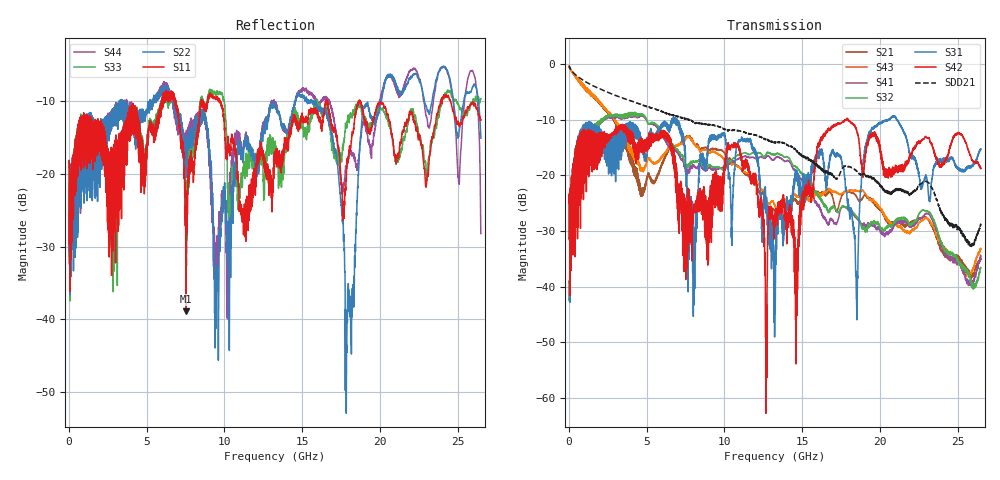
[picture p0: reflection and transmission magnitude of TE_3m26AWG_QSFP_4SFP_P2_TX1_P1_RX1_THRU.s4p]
!Agilent Technologies,N5222A,MY51421691,A.10.00.00
!Agilent N5222A: A.10.00.00
!Date: Friday, January 30, 2015 12:33:28
!Correction: S11(Full 4 Port(1,2,3,4))
!S12(Full 4 Port(1,2,3,4))
!S13(Full 4 Port(1,2,3,4))
!S14(Full 4 Port(1,2,3,4))
!S21(Full 4 Port(1,2,3,4))
!S22(Full 4 Port(1,2,3,4))
!S23(Full 4 Port(1,2,3,4))
!S24(Full 4 Port(1,2,3,4))
!S31(Full 4 Port(1,2,3,4))
!S32(Full 4 Port(1,2,3,4))
!S33(Full 4 Port(1,2,3,4))
!S34(Full 4 Port(1,2,3,4))
!S41(Full 4 Port(1,2,3,4))
!S42(Full 4 Port(1,2,3,4))
!S43(Full 4 Port(1,2,3,4))
!S44(Full 4 Port(1,2,3,4))
!S4P File: Measurements: <S11,S12,S13,S14>,
!<S21,S22,S23,S24>,
!<S31,S32,S33,S34>,
!<S41,S42,S43,S44>:
# Hz S  dB  R 50.0
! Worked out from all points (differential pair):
!   2650 points, 10 MHz to 26.5 GHz, reference 50 ohm
!   strongest paths, dB at 10 MHz, 6.63 GHz, 13.26 GHz, 19.88 GHz, 26.5 GHz:
!     S42: -25.0, -16.1, -29.3, -13.4, -18.7
!     S31: -25.0, -10.4, -36.8, -10.8, -15.2
!     S32: -39.3, -14.4, -16.2, -28.4, -36.6
!     S41: -39.3, -15.0, -17.0, -29.3, -34.6
!     S43: -0.4, -15.0, -25.6, -25.4, -33.3
!     S21: -0.4, -15.1, -26.5, -25.8, -35.1
!   taken as a pair (ports 3,1 in; 4,2 out), SDD21 dB: -0.3, -9.2, -14.1, -21.2, -29.0
!   lowest |S11| = -38.9 dB at 7.52 GHz (marker M1), VSWR 1.02, Z = 51.1 + j0.187 ohm
!   |S11| at or under -10 dB: start of sweep to 5.957 GHz; 9.722 GHz to 16.5 GHz (6.776 GHz wide, 51.7 % of centre); 18.76 GHz to 23.91 GHz (5.153 GHz wide, 24.1 % of centre)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
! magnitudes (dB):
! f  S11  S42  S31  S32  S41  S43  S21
! 10 MHz  -18.2  -25.0  -25.0  -39.3  -39.3  -0.4  -0.4
! 1.7 GHz  -14.1  -12.8  -11.3  -11.6  -11.7  -6.0  -6.1
! 7.52 GHz  -38.9  -38.7  -19.8  -18.2  -19.1  -13.4  -13.1
! 16.45 GHz  -11.0  -13.0  -19.8  -25.1  -27.5  -22.9  -23.2
! 17.9 GHz  -17.9  -9.7  -24.4  -25.8  -26.0  -22.9  -22.9
! 19.08 GHz  -13.3  -16.1  -14.6  -29.8  -29.0  -23.3  -23.5
! 26.5 GHz  -12.6  -18.7  -15.2  -36.6  -34.6  -33.3  -35.1
